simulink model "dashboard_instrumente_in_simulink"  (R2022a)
settings: Solver=ode1  StartTime=0.0  StopTime=inf  FixedStep=1  RelTol=1e-3

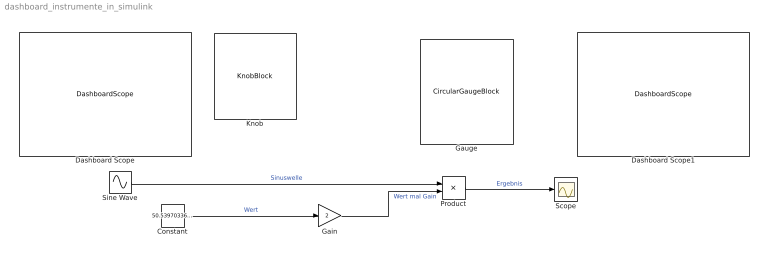
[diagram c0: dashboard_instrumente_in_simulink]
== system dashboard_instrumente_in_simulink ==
  Constant : Constant  Value=50.53970336914062
  Dashboard Scope : DashboardScope
  Dashboard Scope1 : DashboardScope
  Gain : Gain  Gain=2
  Gauge : CircularGaugeBlock
  Knob : KnobBlock
  Product : Product
  Scope : Scope
  Sine Wave : Sin  SampleTime=0
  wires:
  Constant/1 -> Gain/1  "Wert"
  Gain/1 -> Product/2  "Wert mal Gain"
  Sine Wave/1 -> Product/1  "Sinuswelle"
  Product/1 -> Scope/1  "Ergebnis"
